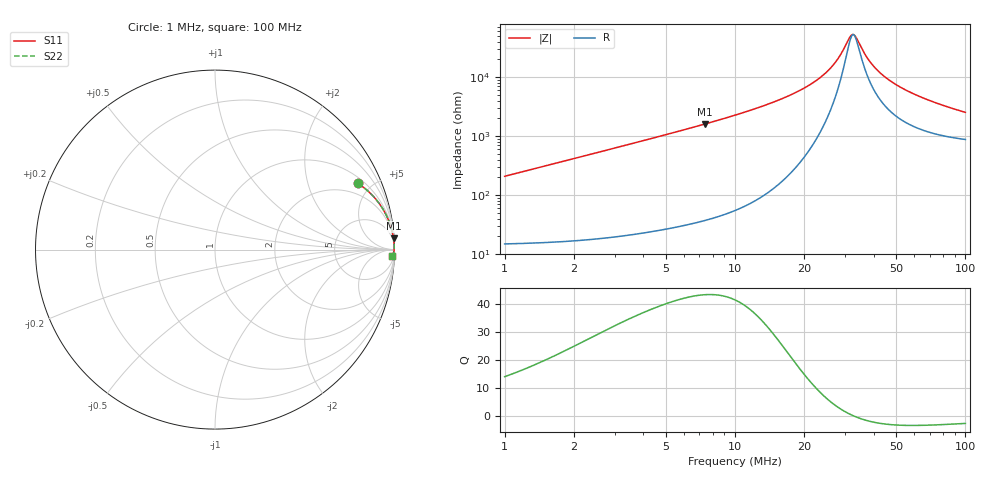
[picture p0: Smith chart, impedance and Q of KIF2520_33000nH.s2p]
!version-2
!date-12.2020
!Series
# MHz S RI R 50
!Freq ReS11 ImS11 ReS21 ImS21 ReS12 ImS12 ReS22 ImS22
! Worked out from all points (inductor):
!   991 points, 1 MHz to 100 MHz, reference 50 ohm
!   read as one part in series: L = 32.9 uH near 1.4 MHz
!   highest Q = 43.3 at 7.4 MHz (marker M1), where L = 34.5 uH
!   self-resonance near 32.6 MHz
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1  0.7956 0.3691  0.2044 -0.3691  0.2044 -0.3691  0.7956 0.3691
2  0.9373 0.2231  0.0627 -0.2231  0.0627 -0.2231  0.9373 0.2231
2.7  0.9641 0.1704  0.0359 -0.1704  0.0359 -0.1704  0.9641 0.1704
3.5  0.978 0.1332  0.022 -0.1332  0.022 -0.1332  0.978 0.1332
5.2  0.9896 0.0898  0.0104 -0.0898  0.0104 -0.0898  0.9896 0.0898
7.4  0.9947 0.062  0.0053 -0.062  0.0053 -0.062  0.9947 0.062
11.1  0.9975 0.0387  0.00249 -0.0387  0.00249 -0.0387  0.9975 0.0387
17.5  0.9987 0.0198  0.00134 -0.0198  0.00134 -0.0198  0.9987 0.0198
22.3  0.9987 0.0116  0.00128 -0.0116  0.00128 -0.0116  0.9987 0.0116
25.8  0.9986 0.00708  0.0014 -0.00708  0.0014 -0.00708  0.9986 0.00708
28.2  0.9985 0.00438  0.00154 -0.00438  0.00154 -0.00438  0.9985 0.00438
31.9  0.9982 0.000716  0.00182 -0.000716  0.00182 -0.000716  0.9982 0.000716
32.8  0.9981 -0.000106  0.0019 0.000106  0.0019 0.000106  0.9981 -0.000106
34  0.998 -0.00117  0.00202 0.00117  0.00202 0.00117  0.998 -0.00117
37  0.9977 -0.00366  0.00233 0.00366  0.00233 0.00366  0.9977 -0.00366
40.3  0.9973 -0.00618  0.00271 0.00618  0.00271 0.00618  0.9973 -0.00618
44.7  0.9967 -0.00928  0.00328 0.00928  0.00328 0.00928  0.9967 -0.00928
50.5  0.9959 -0.013  0.00413 0.013  0.00413 0.013  0.9959 -0.013
57.8  0.9947 -0.0172  0.00535 0.0172  0.00535 0.0172  0.9947 -0.0172
67  0.9929 -0.0221  0.00709 0.0221  0.00709 0.0221  0.9929 -0.0221
83.5  0.9893 -0.0296  0.0107 0.0296  0.0107 0.0296  0.9893 -0.0296
100  0.9851 -0.0361  0.0149 0.0361  0.0149 0.0361  0.9851 -0.0361
